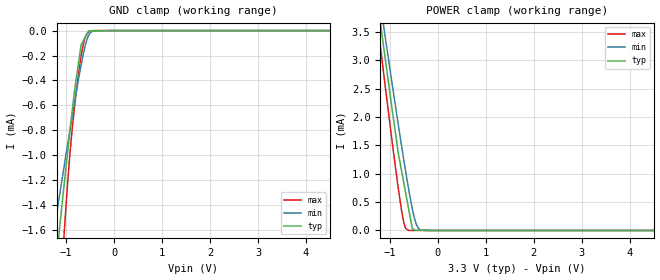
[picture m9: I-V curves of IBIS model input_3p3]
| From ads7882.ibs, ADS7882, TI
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|   input_3p3 Model
[Model]   input_3p3
Model_type   Input
Vinl = 0.8
Vinh = 2.3
|   typ   min   max
|   (nom PVT)   (Fast PVT)   (slow PVT)
|C_comp from frequency sweep method (F=1.5MHz)
|Average
C_comp   2.392e-12   2.313e-12   2.475e-12
|C_comp from LC tank measurement(L=1nH)
|Resonant Frequency(Hz)   3.590e+09   3.640e+09   3.520e+09
|C_comp   1.967e-12   1.914e-12   2.046e-12
| Where nom  PVT is Nominal Process,  3.3V,  25C
|   Fast PVT is Strong Process,   3.6V,  -40C
|   Slow PVT is Weak Process,   3V,  85C
[Model Spec]
Vinh   2.3   2   2.6
[Voltage Range]   3.3   3   3.6
|Ambient Temperature   25   85   -40
|Junction Temperature
[Temperature Range]   25   85   -40
[Power Clamp Reference]   3.3   3   3.6
[GND Clamp Reference]   0   0   0
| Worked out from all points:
|   GND clamp passes 1 mA (typ) near -0.98 V on its own axis
|   POWER clamp passes 1 mA (typ) near -0.74 V on its own axis
[GND Clamp]
|   Voltage   I(typ)   I(min)   I(max)
-3.3V     -9.947mA   -6.818mA   -17.28mA
-1.374V   -2.481mA   -1.911mA   -3.774mA
-1.169V   -1.709mA   -1.399mA   -2.419mA
-1.134V   -1.577mA   -1.313mA   -2.205mA
-1.086V   -1.396mA   -1.196mA   -1.907mA
-1.025V   -1.177mA   -1.049mA   -1.532mA
-877.2mV  -659.2uA   -696.8uA   -803.8uA
-686.4mV  -112.5uA   -275uA     -203.8uA
-614.4mV  -60.8uA    -143.7uA   -71.09uA
-534.6mV  -3.468uA   -41.73uA   -12.16uA
0V        0A         0A         0A
6.6V      0A         0A         0A
[POWER Clamp]
|   Voltage   I(typ)   I(min)   I(max)
-3.3V     17.29mA    16.53mA    18.25mA
-1.259V   4.05mA     4.354mA    3.661mA
-1.161V   3.431mA    3.779mA    2.984mA
-1.129V   3.226mA    3.593mA    2.76mA
-825mV    1.366mA    1.865mA    743.9uA
-754.8mV  1.046mA    1.483mA    345.2uA
-682.8mV  717.1uA    1.101mA    64.91uA
-610.8mV  388.6uA    738.3uA    2.245uA
-534.6mV  40.89uA    390.1uA    1.466uA
-447mV    6.204uA    104uA      570.5nA
-360mV    4.667uA    9.841uA    0A
6.6V      0A         0A         0A
